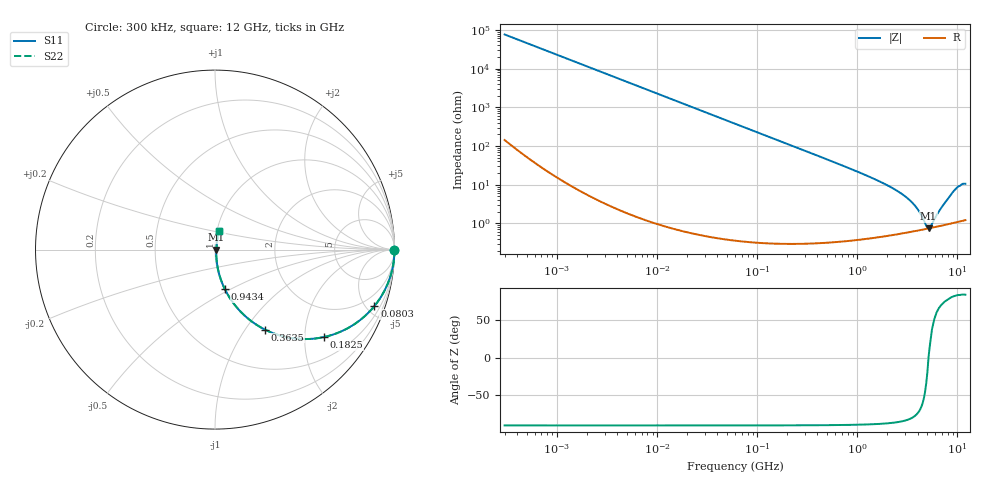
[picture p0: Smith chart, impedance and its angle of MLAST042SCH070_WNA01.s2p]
! MLAST042SCH070_WNA01  S-PARAMETER MODEL  ( General Type )
! Model Generated by TAIYO YUDEN Corporation (http://www.ty-top.com)
! Version 1.0
! TAIYO YUDEN Control No. 150820
! Copyright(c) 2015 TAIYO YUDEN CO.,LTD. All Rights Reserved.
! Product Description (link to TY-COMPAS)
! https://ds.yuden.co.jp/TYCOMPAS/or/detail?pn=MLAST042SCH070BWNA01&u=M
! Products Name : Multilayer Ceramic Capacitors
! Characteristics :
!  Capacitance : 7 pF , Rated Voltage : 25V , TCC : CH / C0H
!  Case Size : 0.4 x 0.2 / 0.016 x 0.008 [mm/inch] , Thickness : 0.2 / 0.008 [mm/inch]
!  (Conditions: Temperature = 25 degC , DC Bias Current/Voltage = 0A / 0V)
! External Node Assignments :
!  1  o---| |---o  2
! GND o---------o GND
! Frequency Range : 0.3MHz  -  12000MHz  [ 401 STEP ]
# MHz S RI R 50
! Freq[MHz].  S11 Real  S11 Imag  S21 Real  S21 Imag  S12 Real  S12 Imag  S22 Real  S22 Imag
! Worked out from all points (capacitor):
!   401 points, 300 kHz to 12 GHz, reference 50 ohm
!   read as one part in series: C = 7.02 pF near 316.3 kHz
!   lowest |Z| = 746 mohm at 5.141 GHz (marker M1)
!   series resonance near 5.138 GHz, so ESL is about 140 pH
!   S11 on the Smith chart (normalised r, x): 300 kHz: open; 80.3 MHz: 1.01, -5.65; 182.5 MHz: 1.01, -2.48; 363.5 MHz: 1.01, -1.24; 943.4 MHz: 1.01, -0.46; 12 GHz: 1.02, +0.21
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0.3  1 -0.00132  4.25e-06 0.00132  4.25e-06 0.00132  1 -0.00132
1.769972  0.9999 -0.0078  6.49e-05 0.0078  6.49e-05 0.0078  0.9999 -0.0078
10.44266  0.9979 -0.046  0.00214 0.046  0.00214 0.046  0.9979 -0.046
27.10171  0.9858 -0.1178  0.0142 0.1178  0.0142 0.1178  0.9858 -0.1178
60  0.9344 -0.2472  0.0656 0.2472  0.0656 0.2472  0.9344 -0.2472
80.29859  0.8883 -0.3145  0.1117 0.3145  0.1117 0.3145  0.8883 -0.3145
182.544  0.606 -0.4874  0.394 0.4874  0.394 0.4874  0.606 -0.4874
353.9943  0.2899 -0.4514  0.7101 0.4514  0.7101 0.4514  0.2899 -0.4514
363.4975  0.2791 -0.4461  0.7209 0.4461  0.7209 0.4461  0.2791 -0.4461
570.2811  0.1357 -0.3384  0.8643 0.3384  0.8643 0.3384  0.1357 -0.3384
943.3804  0.0543 -0.2189  0.9457 0.2189  0.9457 0.2189  0.0543 -0.2189
2088.533  0.0129 -0.0892  0.9871 0.0892  0.9871 0.0892  0.0129 -0.0892
2870.14  0.00847 -0.0538  0.9915 0.0538  0.9915 0.0538  0.00847 -0.0538
3547.679  0.00725 -0.0332  0.9928 0.0332  0.9928 0.0332  0.00725 -0.0332
4050.141  0.007 -0.0211  0.993 0.0211  0.993 0.0211  0.007 -0.0211
4875.354  0.00722 -0.00484  0.9928 0.00484  0.9928 0.00484  0.00722 -0.00484
5140.631  0.0074 4.41e-05  0.9926 -4.41e-05  0.9926 -4.41e-05  0.0074 4.41e-05
5420.343  0.00763 0.00366  0.9924 -0.00366  0.9924 -0.00366  0.00763 0.00366
6699.894  0.00898 0.0206  0.991 -0.0206  0.991 -0.0206  0.00898 0.0206
9207.246  0.0148 0.067  0.9852 -0.067  0.9852 -0.067  0.0148 0.067
10511.28  0.0191 0.0887  0.9809 -0.0887  0.9809 -0.0887  0.0191 0.0887
12000  0.0227 0.1018  0.9773 -0.1018  0.9773 -0.1018  0.0227 0.1018
